(* Logix 5000 Routine export IS7800_Send_Receive_Data; software revision 33.01 *)

VAR_GLOBAL   (* controller tags *)
   Blank : SINT[128];
   Data_From_IS7800 : STRING := '$13$04$00$00$F0I$02$00$10$06$9E?$14$00$00$00Hello PLC. I$'m Job 3$00$00$00$00$00$00$00$00$00$00$00$00$00$00$00$00$00$00$00$00$00$00$00$00$00$00$00$00$00$00$00$00$00$00$00$00$00$00$00$00$00$00$00$00$0;
   IS7800_Send_Data_CMD : BOOL;
   ONS : DINT;
   TimerTriggerCMD : BOOL;
END_VAR

PROGRAM MainProgram

ROUTINE IS7800_Send_Receive_Data   (* ladder *)
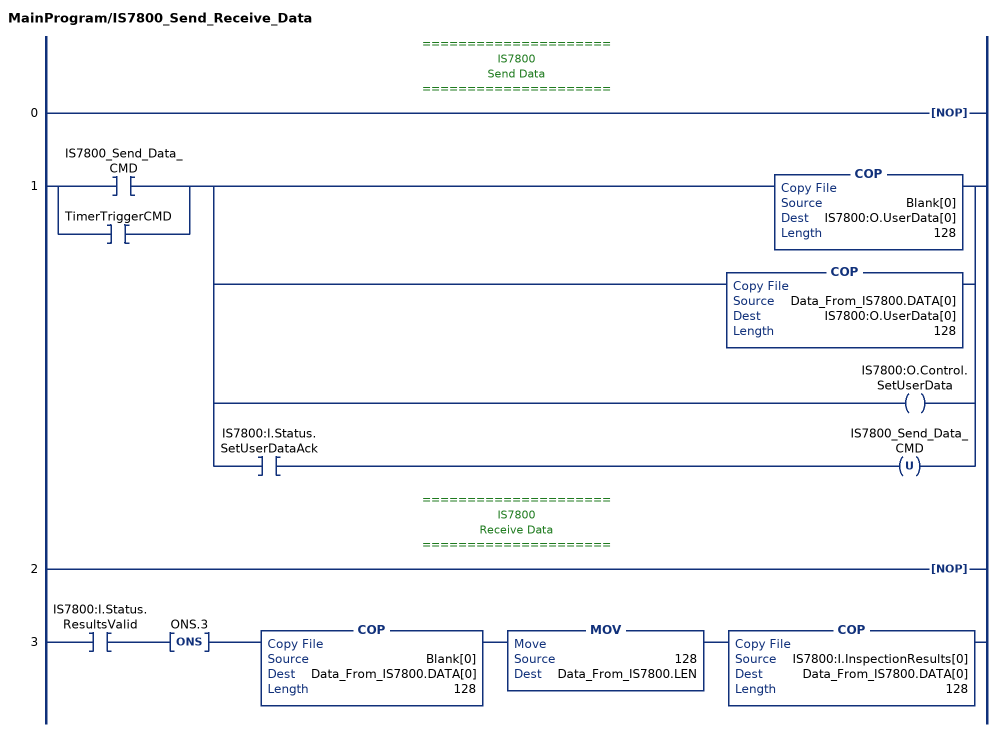
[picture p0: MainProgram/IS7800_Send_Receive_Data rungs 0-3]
   // =====================
   // IS7800
   // Send Data
   // =====================
   0: NOP();
   1: [XIC(IS7800_Send_Data_CMD) ,XIC(TimerTriggerCMD) ][COP(Blank[0],IS7800:O.UserData[0],128) ,COP(Data_From_IS7800.DATA[0],IS7800:O.UserData[0],128) ,OTE(IS7800:O.Control.SetUserData) ,XIC(IS7800:I.Status.SetUserDataAck) OTU(IS7800_Send_Data_CMD) ];
   // =====================
   // IS7800
   // Receive Data
   // =====================
   2: NOP();
   3: XIC(IS7800:I.Status.ResultsValid)ONS(ONS.3)COP(Blank[0],Data_From_IS7800.DATA[0],128)MOV(128,Data_From_IS7800.LEN)COP(IS7800:I.InspectionResults[0],Data_From_IS7800.DATA[0],128);
END_ROUTINE
END_PROGRAM
